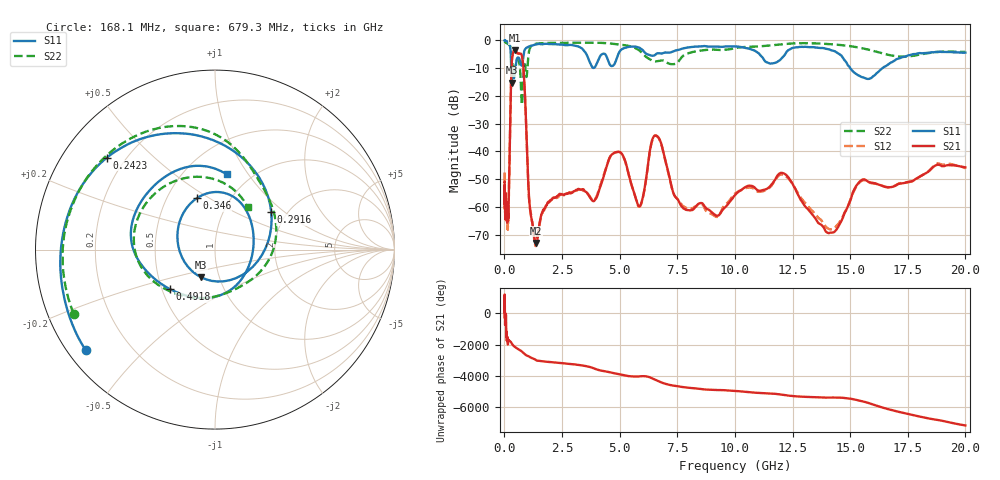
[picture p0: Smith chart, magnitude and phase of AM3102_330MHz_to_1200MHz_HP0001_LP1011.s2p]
! Date/Time: Tue, Sep 11, 2018 5:10 PM
! Network Analyzer: Agilent Technologies E8362B Rev: A.07.50.63
! Sweep from 0.010 to 20.000 GHz, 1601 Points, Sweep Type: LOG
! Power Supply: 4.950 V, 0.001 A
# Hz S DB R 50
!freq MagS11 AngS11 MagS21 AngS21 MagS12 AngS12 MagS22 AngS22
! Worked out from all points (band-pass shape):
!   1601 points, 10 MHz to 20 GHz, reference 50 ohm
!   highest |S21| = -3.50 dB at 447.2 MHz (marker M1); lowest = -73.0 dB at 1.359 GHz (marker M2)
!   |S21| within 3 dB of the highest: 332.5 MHz to 783.4 MHz (450.9 MHz wide, 80.8 % of centre)
!   lowest |S11| = -15.3 dB at 316.2 MHz (marker M3), VSWR 1.42, Z = 40.8 - j12.9 ohm
!   |S11| at or under -10 dB: 295.9 MHz to 351.4 MHz (55.44 MHz wide, 17.1 % of centre); 364.5 MHz to 485.6 MHz (121 MHz wide, 28.5 % of centre); 15.01 GHz to 16.4 GHz (1.394 GHz wide, 8.88 % of centre)
!   |S22| runs from -23.1 to -0.3 dB; largest |S21 - S12| = 0.012
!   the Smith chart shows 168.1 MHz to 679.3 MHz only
!   S11 on the Smith chart (normalised r, x): 168.1 MHz: 0.05, -0.34; 242.3 MHz: 0.13, +0.36; 291.6 MHz: 1.66, +0.81; 346 MHz: 0.70, +0.44; 491.8 MHz: 0.55, -0.27; 679.3 MHz: 0.79, +0.80
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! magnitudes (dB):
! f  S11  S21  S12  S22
! 10 MHz  0.0  -50.9  -47.6  -0.3
! 35.55 MHz  0.0  -61.0  -61.1  -0.5
! 126.4 MHz  -0.4  -63.6  -64.7  -1.1
! 168.1 MHz  -0.8  -63.1  -63.2  -1.3
! 242.3 MHz  -2.0  -34.7  -34.9  -1.8
! 291.6 MHz  -8.5  -14.2  -14.3  -3.6
! 316.2 MHz  -15.3  -8.3  -8.3  -5.9
! 346 MHz  -10.4  -5.7  -5.8  -8.0
! 447.2 MHz  -12.1  -3.5  -3.5  -11.1
! 491.8 MHz  -9.5  -3.7  -3.8  -9.0
! 679.3 MHz  -7.5  -4.7  -4.7  -10.5
! 833.3 MHz  -5.2  -10.8  -10.8  -11.3
! 1.082 GHz  -2.1  -58.0  -58.2  -3.5
! 1.359 GHz  -1.4  -73.0  -73.9  -1.2
! 1.59 GHz  -1.3  -63.2  -63.7  -1.0
! 4.855 GHz  -6.9  -40.2  -40.2  -1.3
! 5.652 GHz  -2.2  -55.5  -55.6  -2.6
! 6.612 GHz  -4.7  -34.4  -34.4  -7.5
! 7.845 GHz  -2.7  -60.9  -60.2  -5.0
! 12.09 GHz  -5.9  -47.8  -48.3  -1.3
! 14.07 GHz  -3.2  -69.4  -67.9  -1.3
! 20 GHz  -4.4  -45.7  -46.0  -4.1
